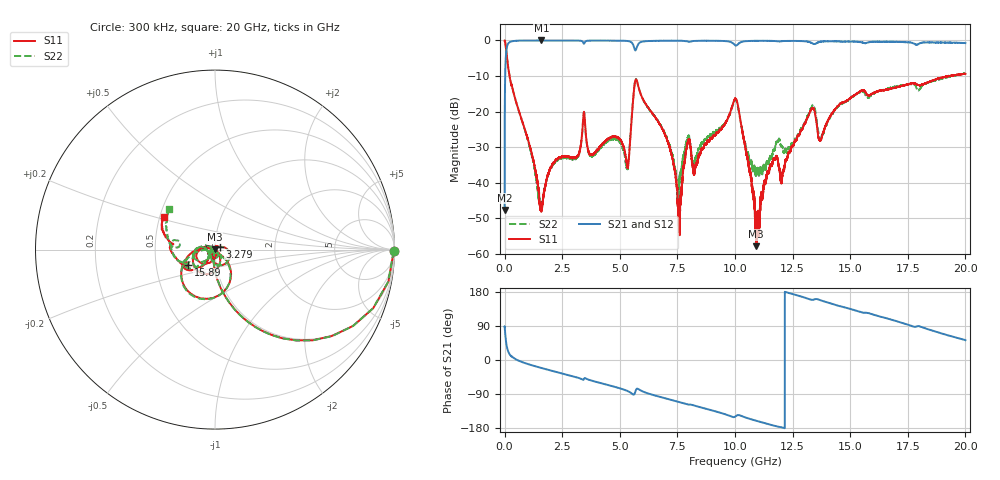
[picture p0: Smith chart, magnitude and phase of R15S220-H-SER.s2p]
!{R15S220}
!Johanson Technology Inc.
!www.johansontechnology.com
!Test Board Conditions:
!Substrate Type  RO4350B
!Substrate Thickness  20 mil
!Substrate Dk  3.66
!TL Type: GCPW
!TL Trace Width  34 mil
!TL Gap  10 mil
!Electrode orientation  Horizontal
!DUT TOPOLOGY	SERIES
!Mounting Pad LxW  26x52 mil
! Created Sat Feb  6 14:21:05 2021
# hz S ma R 50
! 2 Port Network Data from SP1.SP block
! freq  magS11  angS11  magS21  angS21  magS12  angS12  magS22  angS22
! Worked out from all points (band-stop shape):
!   20001 points, 300 kHz to 20 GHz, reference 50 ohm
!   highest |S21| = 0.00 dB at 1.596 GHz (marker M1); lowest = -47.7 dB at 300 kHz (marker M2)
!   |S21| within 3 dB of the highest: 73.1 MHz to end of sweep
!   lowest |S11| = -57.8 dB at 10.92 GHz (marker M3), VSWR 1.00, Z = 49.9 + j0.107 ohm
!   |S11| at or under -10 dB: 214.6 MHz to 19.25 GHz (19.03 GHz wide, 196 % of centre); 19.24955 GHz to 19.2522 GHz (2.646 MHz wide, 0.0137 % of centre); 19.29642 GHz to 19.33254 GHz (36.12 MHz wide, 0.187 % of centre)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
!   |S22| runs from -46.9 to 0.0 dB; largest |S21 - S12| = 0.015
!   S11 on the Smith chart (normalised r, x): 300 kHz: open; 3.279 GHz: 1.05, +0.03; 15.89 GHz: 0.73, -0.13; 20 GHz: 0.53, +0.22
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300000  0.9962 -0.5  0.004136 88.7  0.004085 90.9  0.9953 -0.5
1.023e8  0.5765 -56.0  0.814 33.9  0.8146 33.8  0.5781 -56.0
1.613e8  0.4066 -67.9  0.9105 21.9  0.9111 21.8  0.4087 -67.8
1.5963e9  0.004141 147.4  0.9995 -21.0  0.9984 -21.0  0.004675 -14.0
2.0803e9  0.01825 76.4  0.9979 -28.8  0.9982 -28.9  0.01809 43.9
3.2793e9  0.03018 32.4  0.9919 -48.8  0.9917 -48.7  0.02961 29.3
3.3343e9  0.03891 23.6  0.9858 -50.2  0.9854 -50.2  0.03826 22.5
5.3143e9  0.01801 -123.1  0.9833 -81.3  0.983 -81.3  0.01576 -120.9
5.7183e9  0.2809 -118.1  0.7662 -77.0  0.7664 -77.0  0.2846 -119.1
6.6673e9  0.07252 172.1  0.9893 -96.1  0.9879 -96.1  0.07301 -175.9
7.5883e9  0.002242 -78.3  0.9903 -111.2  0.991 -111.2  0.0115 -60.3
7.9583e9  0.03804 -69.8  0.9666 -117.6  0.9654 -117.5  0.04354 -72.6
8.2643e9  0.01623 -65.3  0.9861 -120.7  0.9871 -120.7  0.02138 -57.0
1.00003e10  0.1516 -121.0  0.8586 -149.9  0.8589 -149.8  0.1452 -124.8
1.09243e10  0.001285 123.1  0.9866 -160.3  0.9854 -160.4  0.01378 165.4
1.15993e10  0.01817 -51.6  0.9852 -171.8  0.9846 -171.8  0.02279 -149.1
1.20513e10  0.01259 -62.5  0.9764 -178.2  0.9784 -178.1  0.03188 -168.5
1.33343e10  0.1098 -140.6  0.919 158.8  0.9198 158.8  0.118 -150.4
1.37373e10  0.0405 -141.0  0.963 157.3  0.9643 157.2  0.042 -153.0
1.58903e10  0.1738 -150.2  0.9536 121.9  0.9535 122.1  0.168 -152.6
1.66673e10  0.2068 -160.2  0.9601 108.4  0.9502 108.4  0.2145 -162.8
2e10  0.3385 147.1  0.9177 52.4  0.9129 52.1  0.3422 138.1
